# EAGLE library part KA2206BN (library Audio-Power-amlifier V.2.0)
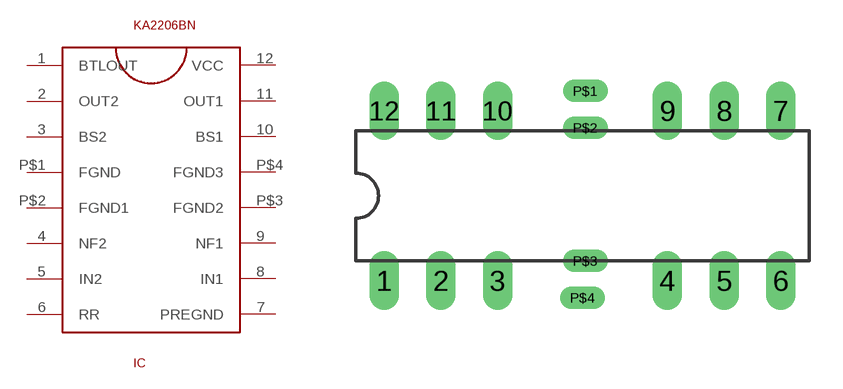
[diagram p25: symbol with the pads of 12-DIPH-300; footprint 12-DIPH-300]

Designator prefix IC

## KA2206BN  [12-DIPH-300]
1  BTLOUT  out
2  OUT2  out
3  BS2
4  NF2
5  IN2  in
6  RR
7  PREGND  pwr
8  IN1  in
9  NF1
10  BS1
11  OUT1  out
12  VCC  pwr
P$1  FGND  pwr
P$2  FGND1  pwr
P$3  FGND2  pwr
P$4  FGND3  pwr

## Footprint 12-DIPH-300 (pad centres in mm)
Dual In Line Package
drill 0.813 long: 1 -8.89,-3.81; 2 -6.35,-3.81; 3 -3.81,-3.81; 4 3.81,-3.81; 5 6.35,-3.81; 6 8.89,-3.81; 7 8.89,3.81; 8 6.35,3.81; 9 3.81,3.81; 10 -3.81,3.81; 11 -6.35,3.81; 12 -8.89,3.81
drill 0.003 pad 1.016 long: P$1 0.127,4.699; P$2 0.127,3.048; P$3 0.127,-2.921; P$4 0,-4.572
